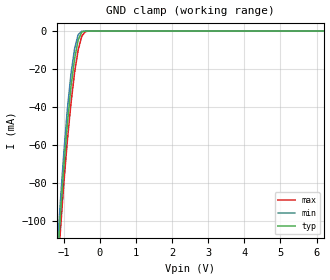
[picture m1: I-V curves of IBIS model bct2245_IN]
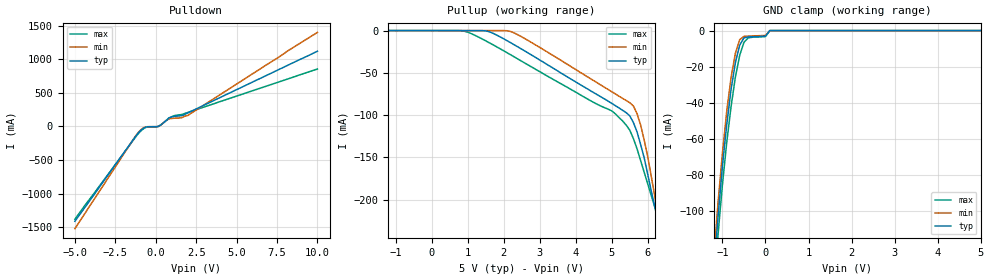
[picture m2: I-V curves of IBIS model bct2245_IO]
| TEXAS INSTRUMENTS INCORPORATED
| Standard Linear and Logic Group
| IBIS Model of SN74BCT2245
| OCTAL TRANSCEIVER AND LINE/MOS DRIVER WITH 3-STATE OUTPUTS
| SOIC 20-pin (DW), SOP 20-pin (NS), SSOP 20-pin (DB), P-DIP 20-pin (N)
[IBIS Ver]   3.2
[Comment Char]  |_char
[File Name]   sn74bct2245.ibs
[File Rev]   3.1
[Date]   Oct.28, 2004
[Source]   File originated at Texas Instruments, Inc.
[Notes]   The following is a sample IBIS file for the BCT2245.
   - FILE REV HISTORY
   - 3.1 Re-Release IBIS file on 10/29/04
   - Power-clamp data deleted as there is no power-clamp diode.
|   - All test data contained in this file are derived from
|   actual measurements.
|   - File created by Nobuhisa Ohtsubo, SLL Product Engineering.
[Disclaimer] Property of Texas Instruments Incorporated.  Unauthorized
   reproduction and/or distribution is strictly prohibited.
   This product is protected under copyright law.
   Created 2000, (C) Copyright 2000, Texas Instruments Inc.,
   All Rights Reserved.
   UNLESS THERE IS A SIGNED, WRITTEN AGREEMENT TO THE
   CONTRARY, TEXAS INSTRUMENTS () IS PROVIDING THE IBIS
   MODELS  AND WITHOUT ANY WARRANTY, EXPRESSED OR
   IMPLIED.  TI assumes no liability for:
   1) the accuracy of the IBIS models provided to your
   company;
   2) the proper functioning of these IBIS Models in your
   design or for any resulting applications; or
   3) infringement of patents, copyrights or intellectual
   property rights resulting from your use of these IBIS
   models.
   TI provides IBIS Models as a service to our customers.
   You and your company shall not distribute, sell or give
   these models to anyone else without prior written
   permission from TI.
   TI reserves the right to make changes to our products or
   to discontinue any semiconductor product or service
   without notice, and advises our customers to obtain the
   latest version of relevant information to verify, before
   placing orders, that the information being relied on is
   current.
   Please be aware that your receipt and use of the IBIS
   information provided shall serve as acceptance of these
   terms and conditions.  If you do not accept these terms,
   you should return or destroy the IBIS models and any
   other accompanying information immediately.
|   Component BCT2245_DW
[Component]   bct2245_DW
[Manufacturer]  Texas Instruments, Inc.
[Package]
|   typ   min   max
R_pkg   0.038   0.033   0.045
L_pkg   5.012nH   4.110nH   6.349nH
C_pkg   0.717pF   0.530pF   0.868pF
[Pin]   signal_name   model_name   R_pin   L_pin   C_pin
1   DIR   bct2245_IN   0.058   5.115nH   0.725pF
2   A1   bct2245_IO   0.053   4.591nH   0.724pF
3   A2   bct2245_IO   0.049   3.754nH   0.572pF
4   A3   bct2245_IO   0.029   2.549nH   0.388pF
5   A4   bct2245_IO   0.031   2.317nH   0.316pF
6   A5   bct2245_IO   0.031   2.317nH   0.316pF
7   A6   bct2245_IO   0.029   2.556nH   0.399pF
8   A7   bct2245_IO   0.049   3.754nH   0.579pF
9   A8   bct2245_IO   0.053   4.591nH   0.724pF
10   GND   GND   0.058   5.115nH   0.725pF
11   B8   bct2245_IO   0.058   5.115nH   0.725pF
12   B7   bct2245_IO   0.053   4.591nH   0.724pF
13   B6   bct2245_IO   0.049   3.754nH   0.579pF
14   B5   bct2245_IO   0.029   2.557nH   0.399pF
15   B4   bct2245_IO   0.031   2.317nH   0.316pF
16   B3   bct2245_IO   0.031   2.317nH   0.316pF
17   B2   bct2245_IO   0.029   2.557nH   0.399pF
18   B1   bct2245_IO   0.049   3.754nH   0.579pF
19   OE_NOT   bct2245_IN   0.053   4.591nH   0.724pF
20   VCC   POWER   0.058   5.115nH   0.725pF
|   Component BCT2245_NS
[Component]   bct2245_NS
[Manufacturer]  Texas Instruments, Inc.
[Package]
|   typ   min   max
R_pkg   0.044   0.029   0.058
L_pkg   3.666nH   2.317nH   5.115nH
C_pkg   0.548pF   0.316pF   0.725pF
[Pin]   signal_name   model_name   R_pin   L_pin   C_pin
1   DIR   bct2245_IN   0.058   5.115nH   0.725pF
2   A1   bct2245_IO   0.053   4.591nH   0.724pF
3   A2   bct2245_IO   0.049   3.754nH   0.572pF
4   A3   bct2245_IO   0.029   2.549nH   0.388pF
5   A4   bct2245_IO   0.031   2.317nH   0.316pF
6   A5   bct2245_IO   0.031   2.317nH   0.316pF
7   A6   bct2245_IO   0.029   2.556nH   0.399pF
8   A7   bct2245_IO   0.049   3.754nH   0.579pF
9   A8   bct2245_IO   0.053   4.591nH   0.724pF
10   GND   GND   0.058   5.115nH   0.725pF
11   B8   bct2245_IO   0.058   5.115nH   0.725pF
12   B7   bct2245_IO   0.053   4.591nH   0.724pF
13   B6   bct2245_IO   0.049   3.754nH   0.579pF
14   B5   bct2245_IO   0.029   2.557nH   0.399pF
15   B4   bct2245_IO   0.031   2.317nH   0.316pF
16   B3   bct2245_IO   0.031   2.317nH   0.316pF
17   B2   bct2245_IO   0.029   2.557nH   0.399pF
18   B1   bct2245_IO   0.049   3.754nH   0.579pF
19   OE_NOT   bct2245_IN   0.053   4.591nH   0.724pF
20   VCC   POWER   0.058   5.115nH   0.725pF
|   Component BCT2245_DB
[Component]   bct2245_DB
[Manufacturer]  Texas Instruments, Inc.
[Package]
|   typ   min   max
R_pkg   0.040   0.035   0.051
L_pkg   3.495nH   3.035nH   4.314nH
C_pkg   0.420pF   0.346pF   0.502pF
[Pin]   signal_name   model_name   R_pin   L_pin   C_pin
1   DIR   bct2245_IN   0.049   4.310nH   0.502pF
2   A1   bct2245_IO   0.048   3.903nH   0.487pF
3   A2   bct2245_IO   0.035   3.189nH   0.396pF
4   A3   bct2245_IO   0.035   3.036nH   0.347pF
5   A4   bct2245_IO   0.035   3.035nH   0.367pF
6   A5   bct2245_IO   0.035   3.035nH   0.367pF
7   A6   bct2245_IO   0.035   3.036nH   0.347pF
8   A7   bct2245_IO   0.035   3.189nH   0.397pF
9   A8   bct2245_IO   0.047   3.899nH   0.488pF
10   GND   GND   0.051   4.314nH   0.500pF
11   B8   bct2245_IO   0.051   4.314nH   0.500pF
12   B7   bct2245_IO   0.047   3.899nH   0.488pF
13   B6   bct2245_IO   0.035   3.189nH   0.397pF
14   B5   bct2245_IO   0.035   3.036nH   0.346pF
15   B4   bct2245_IO   0.035   3.035nH   0.367pF
16   B3   bct2245_IO   0.035   3.035nH   0.367pF
17   B2   bct2245_IO   0.035   3.036nH   0.346pF
18   B1   bct2245_IO   0.035   3.189nH   0.397pF
19   OE_NOT   bct2245_IN   0.047   3.899nH   0.488pF
20   VCC   POWER   0.051   4.314nH   0.502pF
|   Component BCT2245_N
[Component]   bct2245_N
[Manufacturer]   Texas Instruments, Inc.
[Package]
|   typ   min   max
R_pkg   4.300e-02   3.800e-02   5.000e-02
L_pkg   7.384e-09   4.680e-09   1.032e-08
C_pkg   5.100e-13   2.310e-13   8.210e-13
[PIN]   signal_name   model_name   R_pin   L_pin   C_pin
1   DIR   bct2245_IN   4.200e-02   9.427e-09   8.100e-13
2   A1   bct2245_IO   4.600e-02   8.544e-09   4.560e-13
3   A2   bct2245_IO   4.800e-02   7.163e-09   4.350e-13
4   A3   bct2245_IO   4.000e-02   4.825e-09   2.610e-13
5   A4   bct2245_IO   4.000e-02   5.284e-09   6.480e-13
6   A5   bct2245_IO   4.000e-02   4.686e-09   2.320e-13
7   A6   bct2245_IO   4.000e-02   6.359e-09   4.890e-13
8   A7   bct2245_IO   3.800e-02   7.982e-09   4.750e-13
9   A8   bct2245_IO   4.300e-02   9.403e-09   4.750e-13
10   GND   GND   5.000e-02   1.032e-08   8.050e-13
11   B8   bct2245_IO   5.000e-02   1.028e-08   8.100e-13
12   B7   bct2245_IO   4.300e-02   9.383e-09   4.770e-13
13   B6   bct2245_IO   3.800e-02   7.978e-09   4.760e-13
14   B5   bct2245_IO   4.000e-02   6.302e-09   4.920e-13
15   B4   bct2245_IO   4.000e-02   4.680e-09   2.310e-13
16   B3   bct2245_IO   4.000e-02   5.284e-09   6.480e-13
17   B2   bct2245_IO   4.000e-02   4.822e-09   2.610e-13
18   B1   bct2245_IO   4.700e-02   7.118e-09   4.390e-13
19   OE_NOT   bct2245_IN   4.600e-02   8.492e-09   4.610e-13
20   VCC   POWER   4.300e-02   9.348e-09   8.210e-13
| Models and submodels in the file (2): bct2245_IN (Input), bct2245_IO (I/O)
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|   Model BCT2245_IN
[Model]   bct2245_IN
Model_type  Input
Polarity   Inverting
Vinl = 0.8
Vinh = 2.0
| variable   typ   min   max
C_comp   1.33pf   1.00pf   1.66pf
[Temperature Range]   25   0   70
[Voltage Range]   5.0   4.5   5.5
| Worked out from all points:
|   GND clamp passes 1 mA (typ) near -0.51 V on its own axis
[GND Clamp]
|   Voltage   I(typ)   I(min)   I(max)
-5V       -1.42A     -1.52A     -1.36A
-1.2V     -130mA     -122mA     -137mA
-1.1V     -99mA      -91.5mA    -107mA
-1V       -72.2mA    -64.7mA    -80.7mA
-900mV    -49mA      -41.2mA    -57.6mA
-800mV    -29.4mA    -22.6mA    -38.1mA
-700mV    -14.6mA    -9.31mA    -21.8mA
-600mV    -4.72mA    -1.9mA     -9.85mA
-500mV    -558uA     -113uA     -2.67mA
-400mV    -36.2uA    -18.3uA    -295uA
-300mV    -14.5uA    -15.8uA    -26.1uA
10V       227uA      246uA      203uA
|   Model BCT245_IO
[Model]   bct2245_IO
Model_type  I/O
Polarity   Non-Inverting
Enable   Active-Low
Vmeas = 1.5v
Cref = 0pf
Vinl = 0.8
Vinh = 2.0
| variable   typ   min   max
C_comp   5.8pf   4.35pf   7.25pf
[Temperature Range]   25   0   70
[Voltage Range]   5.0   4.5   5.5
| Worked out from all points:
|   slope of the pulldown table from 0 to 0.75 V, typ, clamps not added: 6.38 ohm
|   slope of the pullup table from 0 to 0.75 V, typ, clamps not added: 69.9 kohm
[Pulldown]
|   Voltage   I(typ)   I(min)   I(max)
-5V       -1.41A     -1.52A     -1.38A
-1.3V     -166mA     -159mA     -175mA
-1V       -74.7mA    -67.7mA    -85mA
-700mV    -17.8mA    -12.6mA    -25.7mA
-500mV    -3.99mA    -3.19mA    -6.45mA
200mV     4.56mA     2.81mA     6.64mA
800mV     128mA      114mA      111mA
1.1V      148mA      122mA      158mA
1.6V      161mA      131mA      178mA
2V        204mA      165mA      210mA
10V       1.12A      1.4A       855mA
[Pullup]
|   Voltage   I(typ)   I(min)   I(max)
-5V       88.6nA     5.3nA      1.31uA
800mV     -12.5uA    4.11nA     -103uA
1.5V      -313uA     -18.8uA    -12.1mA
2.2V      -14.5mA    -1.17mA    -28.8mA
5V        -86.2mA    -72.4mA    -95.1mA
5.4V      -97.2mA    -82.8mA    -112mA
5.6V      -109mA     -89.4mA    -128mA
5.7V      -120mA     -98.4mA    -140mA
5.9V      -151mA     -130mA     -168mA
6.3V      -230mA     -222mA     -225mA
6.4V      -249mA     -246mA     -239mA
10V       -956mA     -1.11A     -748mA
[GND Clamp]
|   Voltage   I(typ)   I(min)   I(max)
-5V       -1.41A     -1.52A     -1.38A
-1.2V     -132mA     -125mA     -142mA
-1.1V     -102mA     -94.3mA    -112mA
-1V       -74.7mA    -67.7mA    -85mA
-900mV    -51.8mA    -44.5mA    -61.7mA
-800mV    -32.5mA    -25.9mA    -42.1mA
-700mV    -17.8mA    -12.6mA    -25.7mA
-600mV    -8.08mA    -5.01mA    -13.7mA
-500mV    -3.99mA    -3.19mA    -6.45mA
0V        -3.08mA    -2.68mA    -3.3mA
100mV     3.08uA     2.68uA     3.3uA
5V        12.4uA     10.8uA     15.5uA
[Ramp]
| variable   typ   min   max
dV/dt_r   1.296/1.163n   1.074/1.093n   1.530/1.383n
dV/dt_f   1.872/1.207n   1.656/1.291n   2.094/1.182n
R_load = 50
|   End Component BCT2245
